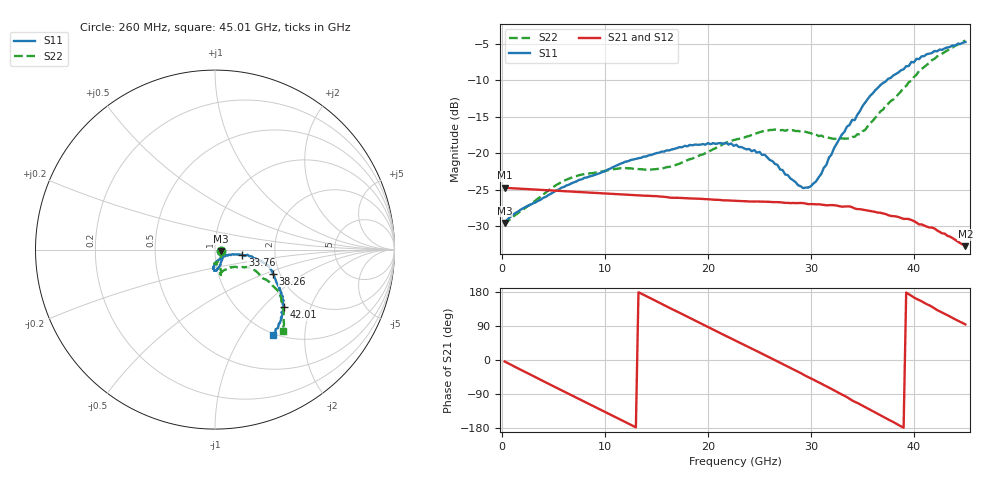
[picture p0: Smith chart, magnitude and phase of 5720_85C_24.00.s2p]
! Device:  ADRF5720
! Description: 0.5dB LSB GaAs MMIC 6-bit Digital Attenuator
! Frequency:  0.000009 -  40 GHz
! Ports:
!	RF1	= Port 1
!	RF2	= Port 2
! Vdd:  3.3 Volt
! Vss:  -3.3 Volt
! Control:  0/3.3 Volt
! State:  24.00 dB attenuation
! Data:  The device was measured using G-S-G Probes on a matrix board.
!  Data was collected using an calibrated 4 port network analyzer.
!  The reference plane for this measurement is at the launchers.
! Note:  Analog Devices supplies this data as a sample of measured data
!  for this product.  Your particular data for this product may vary.
!  Data was taken at 85 degrees C.
!  Analog Devices reserves the right to change this data at anytime.
# GHZ S DB R 45.0
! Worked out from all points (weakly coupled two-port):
!   180 points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, 260 MHz to 45.01 GHz, reference 45 ohm
!   highest |S21| = -24.72 dB at 260 MHz (marker M1); lowest = -32.7 dB at 45.01 GHz (marker M2)
!   lowest |S11| = -29.5 dB at 260 MHz (marker M3), VSWR 1.07, Z = 48 - j0.786 ohm
!   |S11| at or under -10 dB: start of sweep to 37.39 GHz
!   |S22| runs from -29.9 to -4.6 dB; largest |S21 - S12| = 0.00031
!   S11 on the Smith chart (normalised r, x): 260 MHz: 1.07, -0.02; 33.76 GHz: 1.36, -0.09; 38.26 GHz: 1.84, -0.56; 42.01 GHz: 1.57, -1.33; 45.01 GHz: 0.97, -1.39
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0.26  -29.52 -14.2  -24.72 -3.8  -24.72 -3.8  -29.90 -15.9
1.26  -28.21 -3.9  -24.81 -17.9  -24.80 -17.9  -28.48 -13.1
5.01  -25.32 -37.4  -25.10 -69.3  -25.09 -69.2  -24.59 -63.2
7.76  -23.57 -52.6  -25.33 -106.6  -25.32 -106.5  -22.93 -80.4
11.51  -21.44 -68.3  -25.64 -157.3  -25.63 -157.2  -22.05 -92.4
15.26  -19.92 -78.0  -25.91 151.3  -25.90 151.5  -22.12 -87.7
18.26  -18.86 -84.6  -26.18 111.0  -26.16 111.1  -20.82 -78.8
22.76  -18.84 -92.3  -26.51 50.1  -26.50 50.2  -18.11 -74.3
25.51  -20.20 -93.1  -26.62 13.2  -26.61 13.4  -16.91 -77.3
29.26  -24.77 -59.8  -26.82 -38.3  -26.80 -38.0  -17.04 -78.2
30.26  -24.12 -41.1  -26.96 -51.9  -26.94 -51.6  -17.48 -77.2
31.01  -22.83 -24.1  -27.03 -62.6  -27.01 -62.3  -17.59 -74.2
33.01  -17.44 -11.4  -27.31 -91.0  -27.28 -90.8  -17.97 -61.2
33.76  -16.14 -11.6  -27.27 -102.3  -27.25 -102.0  -18.01 -53.5
34.76  -14.26 -10.8  -27.65 -116.7  -27.65 -116.5  -17.42 -45.9
35.76  -12.15 -13.3  -27.90 -131.2  -27.89 -131.0  -15.89 -38.0
37.76  -9.70 -19.1  -28.57 -160.4  -28.54 -160.1  -12.86 -27.8
38.26  -9.16 -22.5  -28.64 -167.6  -28.61 -167.1  -12.32 -27.3
40.51  -7.14 -34.0  -29.73 158.3  -29.70 158.8  -8.75 -30.9
42.01  -6.02 -39.5  -30.29 136.2  -30.29 136.6  -7.09 -35.1
43.51  -5.48 -45.8  -31.41 114.6  -31.37 115.2  -5.68 -42.6
45.01  -4.79 -56.1  -32.71 93.9  -32.67 94.2  -4.58 -50.3
